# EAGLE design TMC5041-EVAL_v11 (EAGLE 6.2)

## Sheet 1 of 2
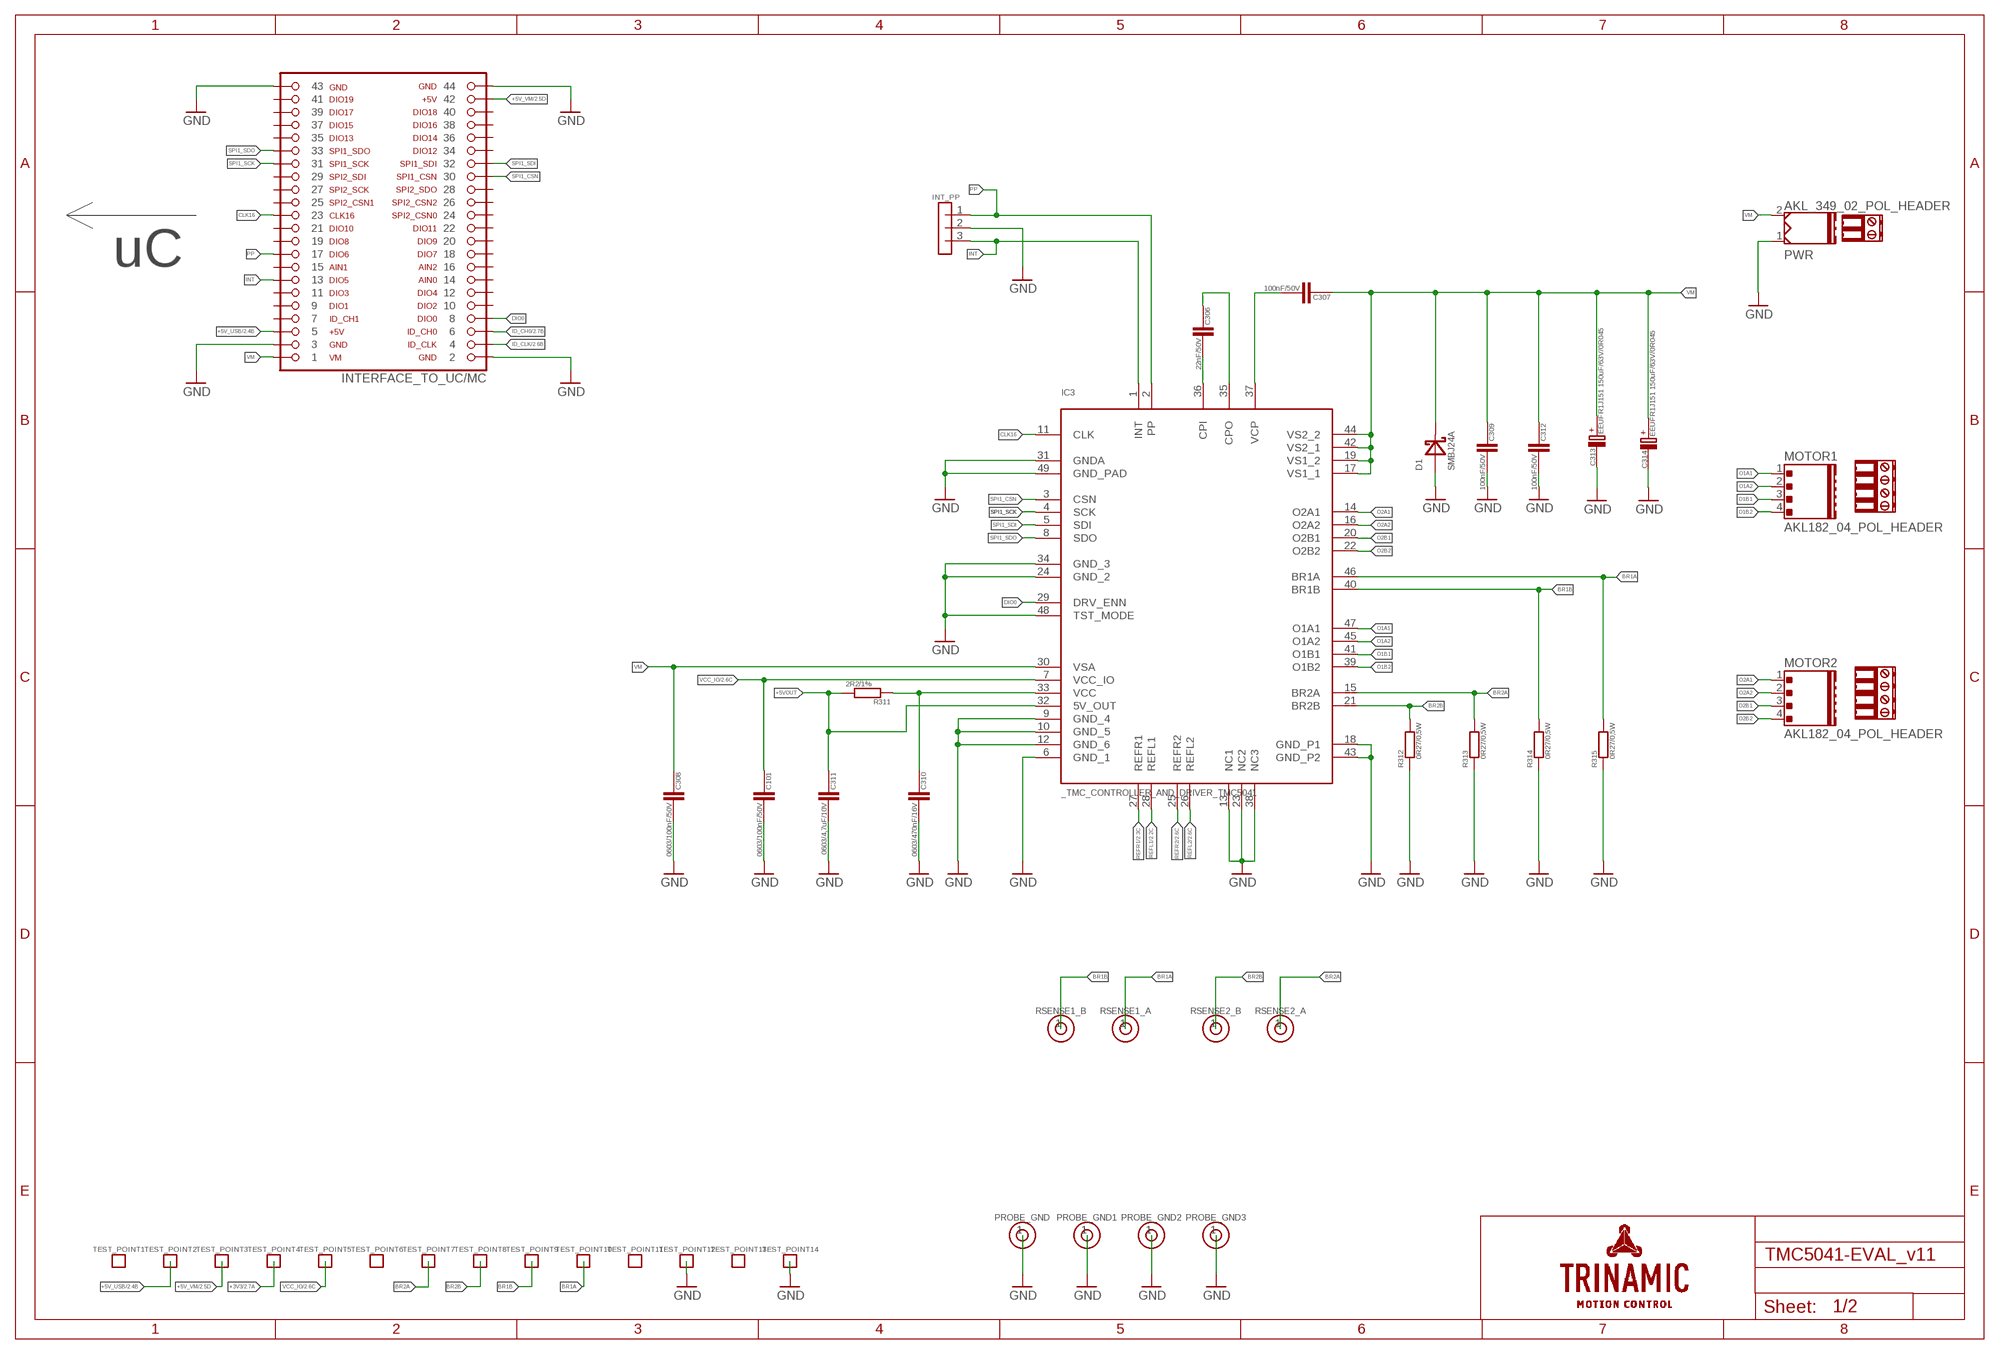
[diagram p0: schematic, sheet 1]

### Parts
C101  0603/100nF/50V  C/0603  [0603]
C306  22nF/50V  C/0603  [0603]
C307  100nF/50V  C/0603  [0603]
C308  0603/100nF/50V  C/0603  [0603]
C309  100nF/50V  C/0603  [0603]
C310  0603/470nF/16V  C/0603  [0603]
C311  0603/4,7uF/10V  C/0603  [0603]
C312  100nF/50V  C/0603  [0603]
C313  EEUFR1J151 150uF/63V/0R045  C_POL5X10X17.5  [C_POL_RAD_THT_5X10]
C314  EEUFR1J151 150uF/63V/0R045  C_POL5X10X17.5  [C_POL_RAD_THT_5X10]
D1  SMBJ24A  SMBJ  [SMB]
IC3  _TMC_CONTROLLER_AND_DRIVER_TMC5041  [_TMC_CONTROLLER_AND_DRIVER_QFN48]
INT_PP  MALE HEADER 2.54  3PIN_1ROWTHT  [3PIN_1ROW_2,54_THT]
INTERFACE_TO_UC/MC  FEMALE_HEADER_SMD_2.54_44_PINSHORTPADS_HOLES  [FEMALE_HEADER_SMD_254_44_PIN_SHORTPADS_HOLES]
MOTOR1  AKL182_04_POL_HEADER  [AKL169_04_POL]
MOTOR2  AKL182_04_POL_HEADER  [AKL169_04_POL]
PROBE_GND  NOT ASSEMBLED  1PIN_1ROW  [1PIN_1ROW_THT]
PROBE_GND1  NOT ASSEMBLED  1PIN_1ROW  [1PIN_1ROW_THT]
PROBE_GND2  NOT ASSEMBLED  1PIN_1ROW  [1PIN_1ROW_THT]
PROBE_GND3  NOT ASSEMBLED  1PIN_1ROW  [1PIN_1ROW_THT]
PWR  AKL_349_02_POL_HEADER  [AKL349_02_POL]
R311  2R2/1%  R/0603  [0603]
R312  0R27/0,5W  R  [1206]
R313  0R27/0,5W  R  [1206]
R314  0R27/0,5W  R  [1206]
R315  0R27/0,5W  R  [1206]
RSENSE1_A  NOT ASSEMBLED  1PIN_1ROW  [1PIN_1ROW_THT]
RSENSE1_B  NOT ASSEMBLED  1PIN_1ROW  [1PIN_1ROW_THT]
RSENSE2_A  NOT ASSEMBLED  1PIN_1ROW  [1PIN_1ROW_THT]
RSENSE2_B  NOT ASSEMBLED  1PIN_1ROW  [1PIN_1ROW_THT]
TERM1  AKL182_04_POL_TERMINAL  [EXTRA_TERMINAL]
TERM2  AKL182_04_POL_TERMINAL  [EXTRA_TERMINAL]
TERM3  AKL_330_2_POL_TERMINAL  [EXTRA_TERMINAL]
TEST_POINT1  NOT ASSEMBLED  PAD_ROUND  [PAD_R1.2]
TEST_POINT2  NOT ASSEMBLED  PAD_ROUND  [PAD_R1.2]
TEST_POINT3  NOT ASSEMBLED  PAD_ROUND  [PAD_R1.2]
TEST_POINT4  NOT ASSEMBLED  PAD_ROUND  [PAD_R1.2]
TEST_POINT5  NOT ASSEMBLED  PAD_ROUND  [PAD_R1.2]
TEST_POINT6  NOT ASSEMBLED  PAD_ROUND  [PAD_R1.2]
TEST_POINT7  NOT ASSEMBLED  PAD_ROUND  [PAD_R1.2]
TEST_POINT8  NOT ASSEMBLED  PAD_ROUND  [PAD_R1.2]
TEST_POINT9  NOT ASSEMBLED  PAD_ROUND  [PAD_R1.2]
TEST_POINT10  NOT ASSEMBLED  PAD_ROUND  [PAD_R1.2]
TEST_POINT11  NOT ASSEMBLED  PAD_ROUND  [PAD_R1.2]
TEST_POINT12  NOT ASSEMBLED  PAD_ROUND  [PAD_R1.2]
TEST_POINT13  NOT ASSEMBLED  PAD_ROUND  [PAD_R1.2]
TEST_POINT14  NOT ASSEMBLED  PAD_ROUND  [PAD_R1.2]

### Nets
+3V3: TEST_POINT4.P$1 ; also sheet 2
+5V_USB: INTERFACE_TO_UC/MC.5 TEST_POINT2.P$1 ; also sheet 2
+5V_VM: INTERFACE_TO_UC/MC.42 TEST_POINT3.P$1 ; also sheet 2
+5VOUT: C311.2 IC3.32(5V_OUT) R311.2
BR1A: IC3.46(BR1A) R315.2 RSENSE1_A.1 TEST_POINT10.P$1
BR1B: IC3.40(BR1B) R314.2 RSENSE1_B.1 TEST_POINT9.P$1
BR2A: IC3.15(BR2A) R313.2 RSENSE2_A.1 TEST_POINT7.P$1
BR2B: IC3.21(BR2B) R312.2 RSENSE2_B.1 TEST_POINT8.P$1
CLK16: IC3.11(CLK) INTERFACE_TO_UC/MC.23
CPI: C306.1 IC3.36(CPI)
CPO: C306.2 IC3.35(CPO)
DIO0: IC3.29(DRV_ENN) INTERFACE_TO_UC/MC.8
GND: C101.1 C308.1 C309.1 C310.1 C311.1 C312.1 C313.- C314.- D1.A IC3.6(GND_1) IC3.9(GND_4) IC3.10(GND_5) IC3.12(GND_6) IC3.13(NC1) IC3.18(GND_P1) IC3.23(NC2) IC3.24(GND_2) IC3.31(GNDA) IC3.34(GND_3) IC3.38(NC3) IC3.43(GND_P2) IC3.48(TST_MODE) IC3.49(GND_PAD) INT_PP.2 INTERFACE_TO_UC/MC.2 INTERFACE_TO_UC/MC.3 INTERFACE_TO_UC/MC.43 INTERFACE_TO_UC/MC.44 PROBE_GND1.1 PROBE_GND2.1 PROBE_GND3.1 PROBE_GND.1 PWR.1 R312.1 R313.1 R314.1 R315.1 TEST_POINT12.P$1 TEST_POINT14.P$1 ; also sheet 2
ID_CH0: INTERFACE_TO_UC/MC.6 ; also sheet 2
ID_CLK: INTERFACE_TO_UC/MC.4 ; also sheet 2
INT: IC3.1(INT) INT_PP.3 INTERFACE_TO_UC/MC.13
O1A1: IC3.47(O1A1) MOTOR1.1
O1A2: IC3.45(O1A2) MOTOR1.2
O1B1: IC3.41(O1B1) MOTOR1.3
O1B2: IC3.39(O1B2) MOTOR1.4
O2A1: IC3.14(O2A1) MOTOR2.1
O2A2: IC3.16(O2A2) MOTOR2.2
O2B1: IC3.20(O2B1) MOTOR2.3
O2B2: IC3.22(O2B2) MOTOR2.4
PP: IC3.2(PP) INT_PP.1 INTERFACE_TO_UC/MC.17
REFL1: IC3.28(REFL1) ; also sheet 2
REFL2: IC3.26(REFL2) ; also sheet 2
REFR1: IC3.27(REFR1) ; also sheet 2
REFR2: IC3.25(REFR2) ; also sheet 2
SPI1_CSN: IC3.3(CSN) INTERFACE_TO_UC/MC.30
SPI1_SCK: IC3.4(SCK) INTERFACE_TO_UC/MC.31
SPI1_SDI: IC3.5(SDI) INTERFACE_TO_UC/MC.32
SPI1_SDO: IC3.8(SDO) INTERFACE_TO_UC/MC.33
VCC: C310.2 IC3.33(VCC) R311.1
VCC_IO: C101.2 IC3.7(VCC_IO) TEST_POINT5.P$1 ; also sheet 2
VCP: C307.1 IC3.37(VCP)
VM: C307.2 C308.2 C309.2 C312.2 C313.+ C314.+ D1.C IC3.17(VS1_1) IC3.19(VS1_2) IC3.30(VSA) IC3.42(VS2_1) IC3.44(VS2_2) INTERFACE_TO_UC/MC.1 PWR.2
Unconnected: INTERFACE_TO_UC/MC.7 INTERFACE_TO_UC/MC.9 INTERFACE_TO_UC/MC.10 INTERFACE_TO_UC/MC.11 INTERFACE_TO_UC/MC.12 INTERFACE_TO_UC/MC.14 INTERFACE_TO_UC/MC.15 INTERFACE_TO_UC/MC.16 INTERFACE_TO_UC/MC.18 INTERFACE_TO_UC/MC.19 INTERFACE_TO_UC/MC.20 INTERFACE_TO_UC/MC.21 INTERFACE_TO_UC/MC.22 INTERFACE_TO_UC/MC.24 INTERFACE_TO_UC/MC.25 INTERFACE_TO_UC/MC.26 INTERFACE_TO_UC/MC.27 INTERFACE_TO_UC/MC.28 INTERFACE_TO_UC/MC.29 INTERFACE_TO_UC/MC.34 INTERFACE_TO_UC/MC.35 INTERFACE_TO_UC/MC.36 INTERFACE_TO_UC/MC.37 INTERFACE_TO_UC/MC.38 INTERFACE_TO_UC/MC.39 INTERFACE_TO_UC/MC.40 INTERFACE_TO_UC/MC.41 TEST_POINT1.P$1 TEST_POINT6.P$1 TEST_POINT11.P$1 TEST_POINT13.P$1

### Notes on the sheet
- uC

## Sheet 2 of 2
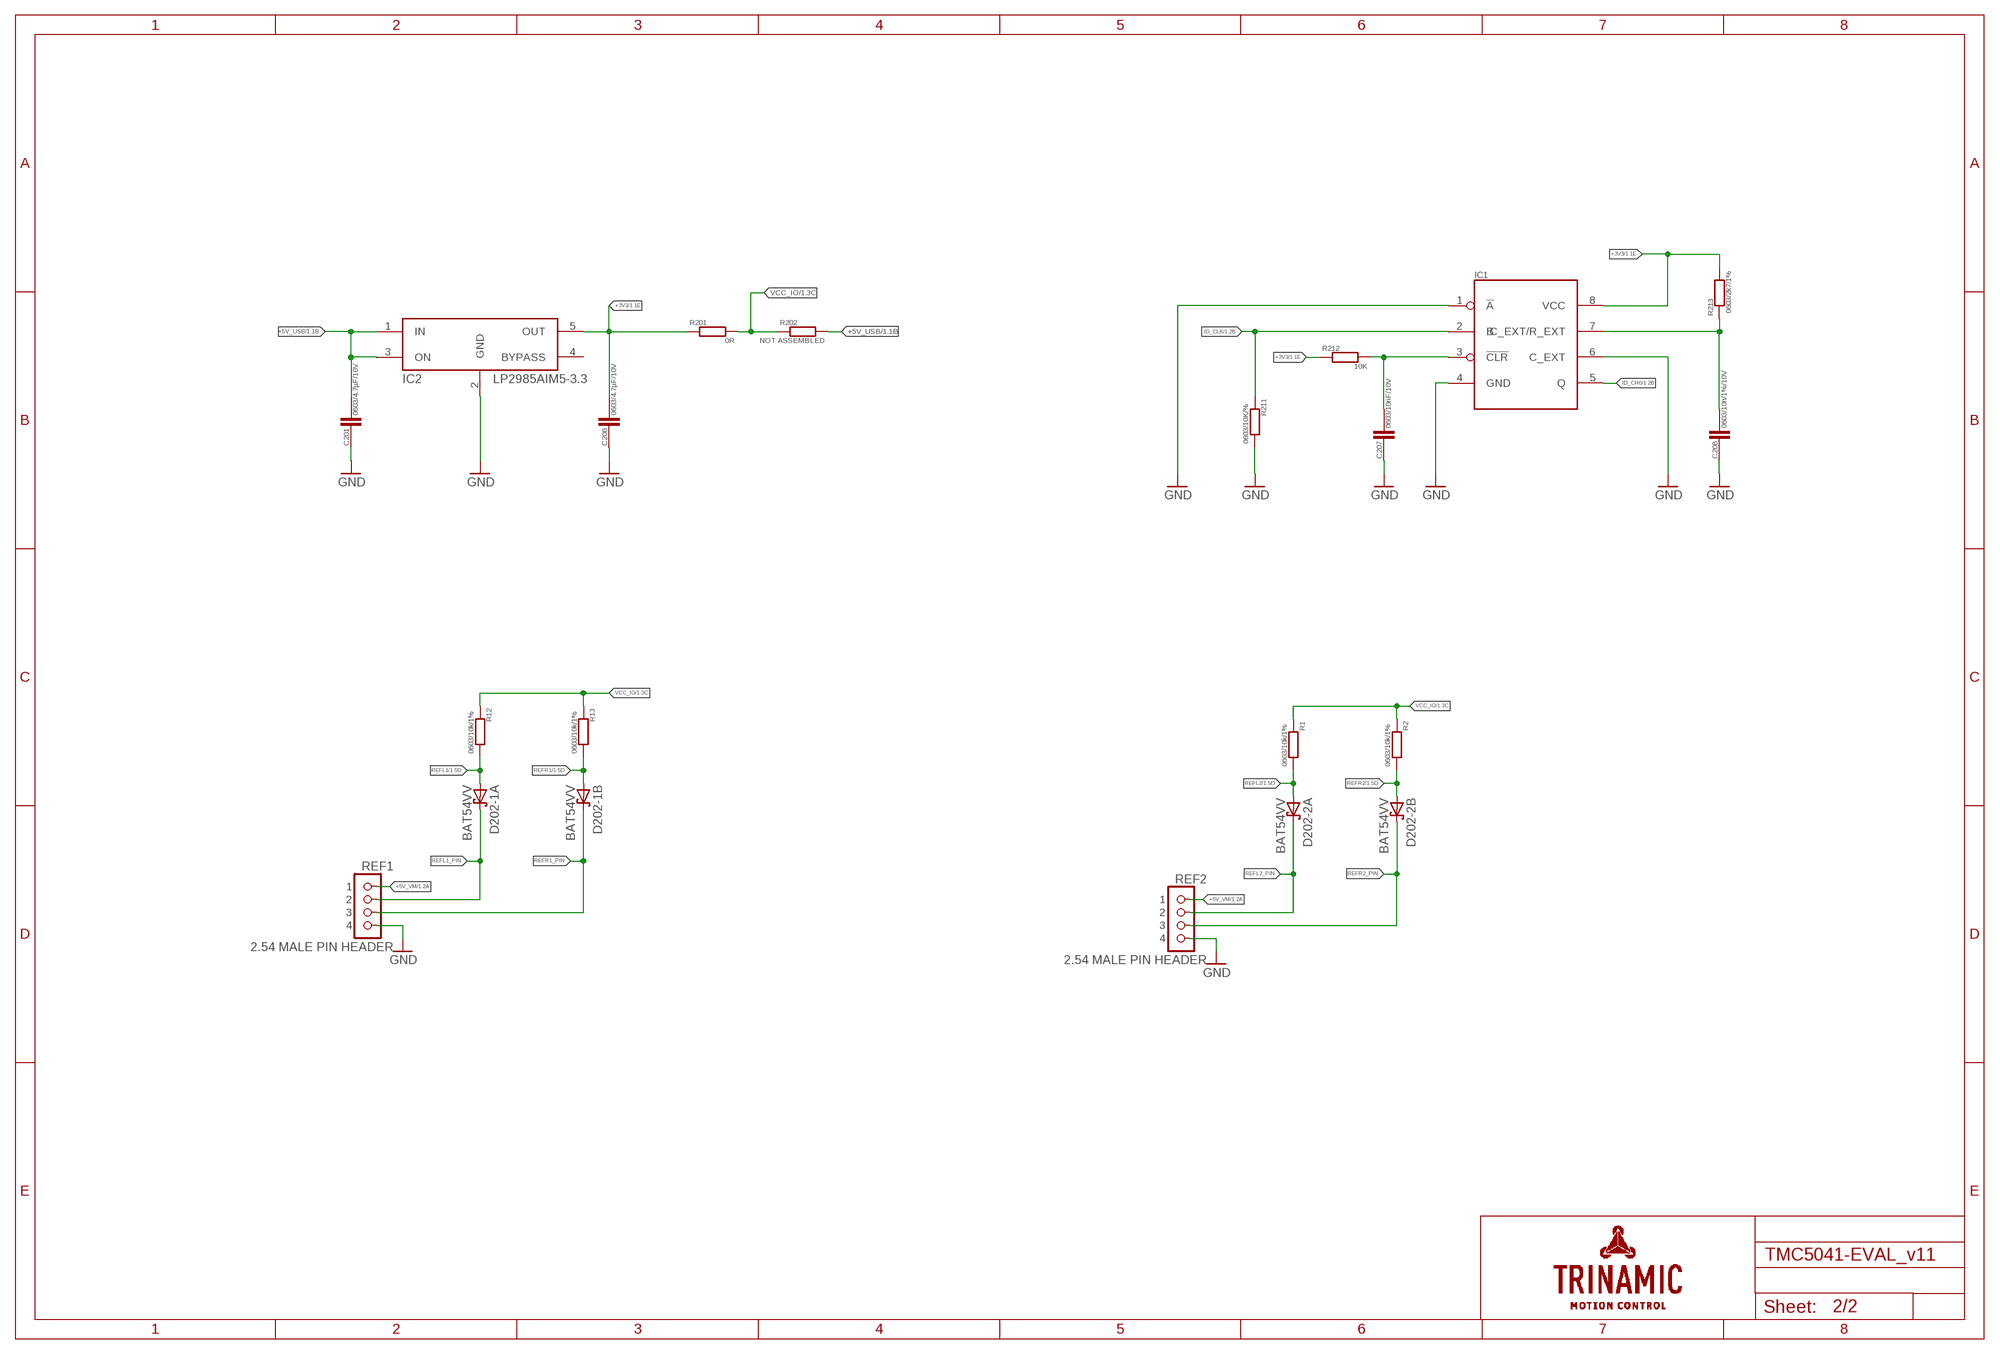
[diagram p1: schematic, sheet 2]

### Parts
C201  0603/4.7µF/10V  RCL_C/0603  [RCL_0603]
C206  0603/4.7µF/10V  RCL_C/0603  [RCL_0603]
C207  0603/10nF/10V  RCL_C/0603  [RCL_0603]
C208  0603/10n/1%/10V  RCL_C/0603  [RCL_0603]
D202-1  BAT54VV  BAS70VV  [SOT666]
D202-2  BAT54VV  BAS70VV  [SOT666]
IC1  SN74LVC1G123DCTR  [SN74LVC1G123DCTR]
IC2  LP2985AIM5-3.3  [SOT23-5]
R1  0603/10k/1%  R/0603  [0603]
R2  0603/10k/1%  R/0603  [0603]
R12  0603/10k/1%  R/0603  [0603]
R13  0603/10k/1%  R/0603  [0603]
R201  0R  R/0603  [0603]
R202  NOT ASSEMBLED  R/0603  [0603]
R211  0603/10K/%  RCL_R/0603  [RCL_0603]
R212  10K  RCL_R/0603  [RCL_0603]
R213  0603/2k7/1%  RCL_R/0603  [RCL_0603]
REF1  2.54 MALE PIN HEADER  4PIN_1ROWTHT  [4PIN_1ROW_2.54_THT]
REF2  2.54 MALE PIN HEADER  4PIN_1ROWTHT  [4PIN_1ROW_2.54_THT]

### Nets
+3V3: C206.1 IC1.8(VCC) IC2.5(OUT) R201.1 R212.1 R213.2 ; also sheet 1
+5V_USB: C201.1 IC2.1(IN) IC2.3(ON) R202.2 ; also sheet 1
+5V_VM: REF1.1 REF2.1 ; also sheet 1
GND: C201.2 C206.2 C207.2 C208.2 IC1.1(!A) IC1.4(GND) IC1.6(C_EXT) IC2.2(GND) R211.2 REF1.4 REF2.4 ; also sheet 1
ID_CH0: IC1.5(Q) ; also sheet 1
ID_CLK: IC1.2(B) R211.1 ; also sheet 1
N$1: C207.1 IC1.3(!CLR) R212.2
N$2: C208.1 IC1.7(C_EXT/R_EXT) R213.1
REFL1: D202-1.1(A:A) R12.2 ; also sheet 1
REFL1_PIN: D202-1.6(A:C) REF1.2
REFL2: D202-2.1(A:A) R1.2 ; also sheet 1
REFL2_PIN: D202-2.6(A:C) REF2.2
REFR1: D202-1.2(B:A) R13.2 ; also sheet 1
REFR1_PIN: D202-1.5(B:C) REF1.3
REFR2: D202-2.2(B:A) R2.2 ; also sheet 1
REFR2_PIN: D202-2.5(B:C) REF2.3
VCC_IO: R1.1 R2.1 R12.1 R13.1 R201.2 R202.1 ; also sheet 1
Unconnected: D202-1.3(C:A) D202-1.4(C:C) D202-2.3(C:A) D202-2.4(C:C) IC2.4(BYPASS)

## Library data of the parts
C101 C306-C312 = _TMC_TE_RCL:C
C201 C206-C208 = TMC_EVAL_driver_TE_v01:RCL_C
C313 C314 = _TMC_TE_RCL:C_POL
D1 = _TMC_TE_D:SMBJ
D202-1 D202-2 = diode:BAS70VV: Silicon Schottky Diodes General-purpose diode for high-speed switching Source: BAS70_1PS7XSB70_SER_8.pdf
IC1 = TMC_EVAL_driver_TE_v01:SN74LVC1G123DCTR
IC2 = TMC_EVAL_driver_TE_v01:LP2985AIM5-3.3
IC3 = TMC5041:_TMC_CONTROLLER_AND_DRIVER_TMC5041
INT_PP = _TMC_TE_con:3PIN_1ROW
INTERFACE_TO_UC/MC = _TMC_TE_con:FEMALE_HEADER_SMD_2.54_44_PIN; 1_PARTNUMBER: 098-3-044-1-NFX-YT0; 1_SUPPLIER: MPE Garry; 2_PARTNUMBER: HLE-122-02-F-DV; 2_SUPPLIER: Samtec
MOTOR1 MOTOR2 = _TMC_TE_con:AKL182_04_POL_HEADER: AKL header, shrouted, 4 pins; 1_PARTNUMBER: 31182104; 1_SUPPLIER: RIA CONNECT; 2_PARTNUMBER: AKL 182-04; 2_SUPPLIER: Reichelt
PROBE_GND PROBE_GND1-PROBE_GND3 RSENSE1_A RSENSE1_B RSENSE2_A RSENSE2_B = _TMC_TE_con:1PIN_1ROW
PWR = _TMC_TE_con:AKL_349_02_POL_HEADER: AKL header, shrouted, 2 pins; 1_PARTNUMBER: 31330102; 1_SUPPLIER: RIA CONNECT; 2_PARTNUMBER: AKL 330-02; 2_SUPPLIER: REICHELT
R1 R2 R12 R13 R201 R202 R311-R315 = _TMC_TE_RCL:R
R211-R213 = TMC_EVAL_driver_TE_v01:RCL_R
REF1 REF2 = _TMC_TE_con:4PIN_1ROW
TERM1 TERM2 = _TMC_TE_con:AKL182_04_POL_TERMINAL: AKL terminal, 4 pins; 1_PARTNUMBER: 31169104; 1_SUPPLIER: RIA CONNECT; 2_PARTNUMBER: AKL 169-04; 2_SUPPLIER: Reichelt
TERM3 = _TMC_TE_con:AKL_330_2_POL_TERMINAL: AKL terminal, 2 pins; 1_PARTNUMBER: 31349102; 1_SUPPLIER: RIA CONNECT; 2_PARTNUMBER: AKL 349-02; 2_SUPPLIER: Reichelt
TEST_POINT1-TEST_POINT14 = _TMC_TE_PADS:PAD_ROUND

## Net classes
0 default: width 0.254 mm, drill 0.15 mm

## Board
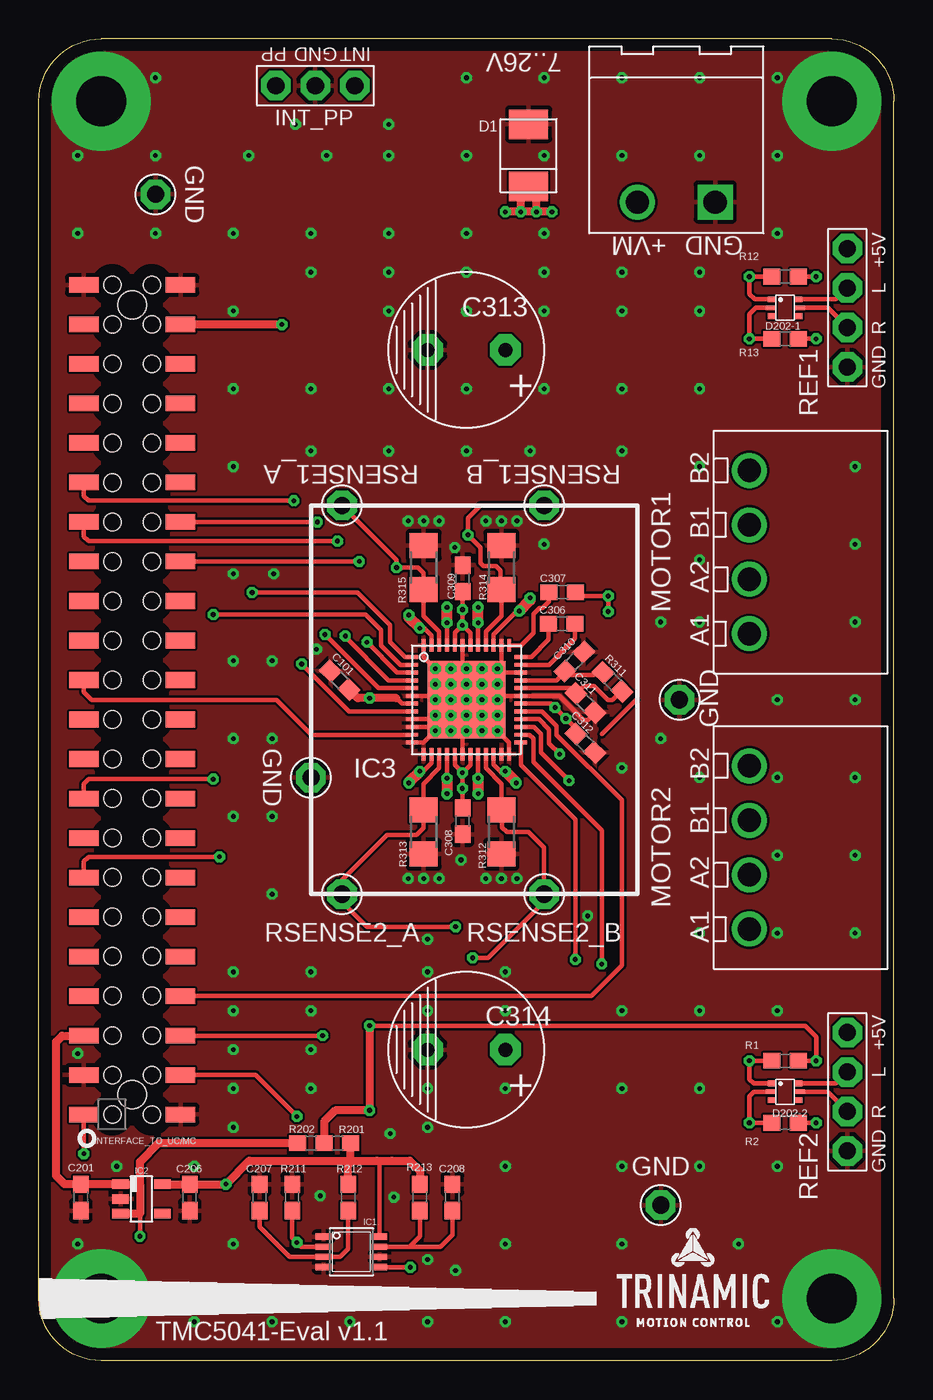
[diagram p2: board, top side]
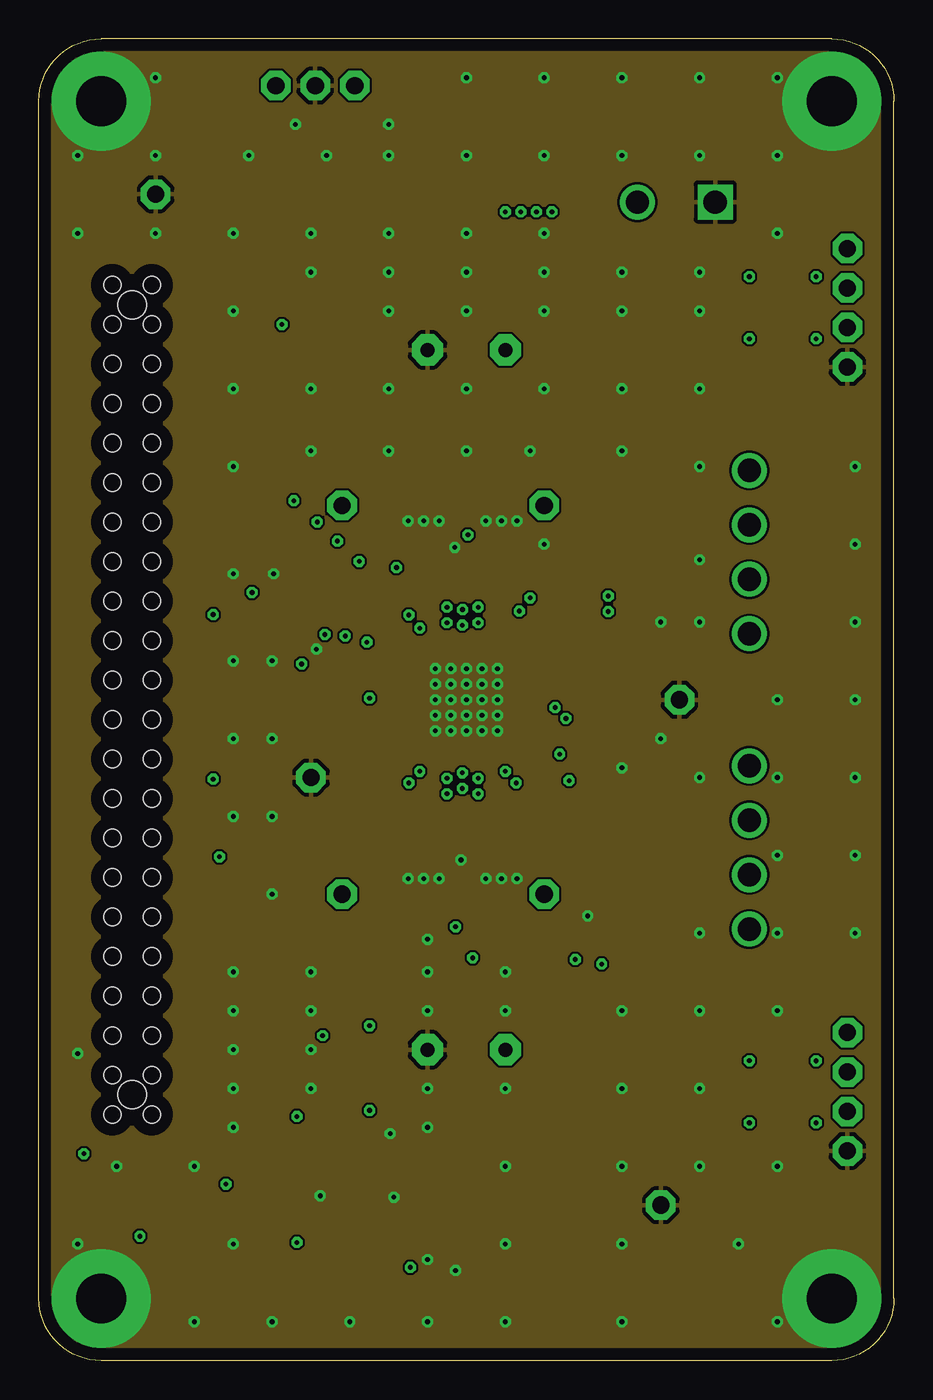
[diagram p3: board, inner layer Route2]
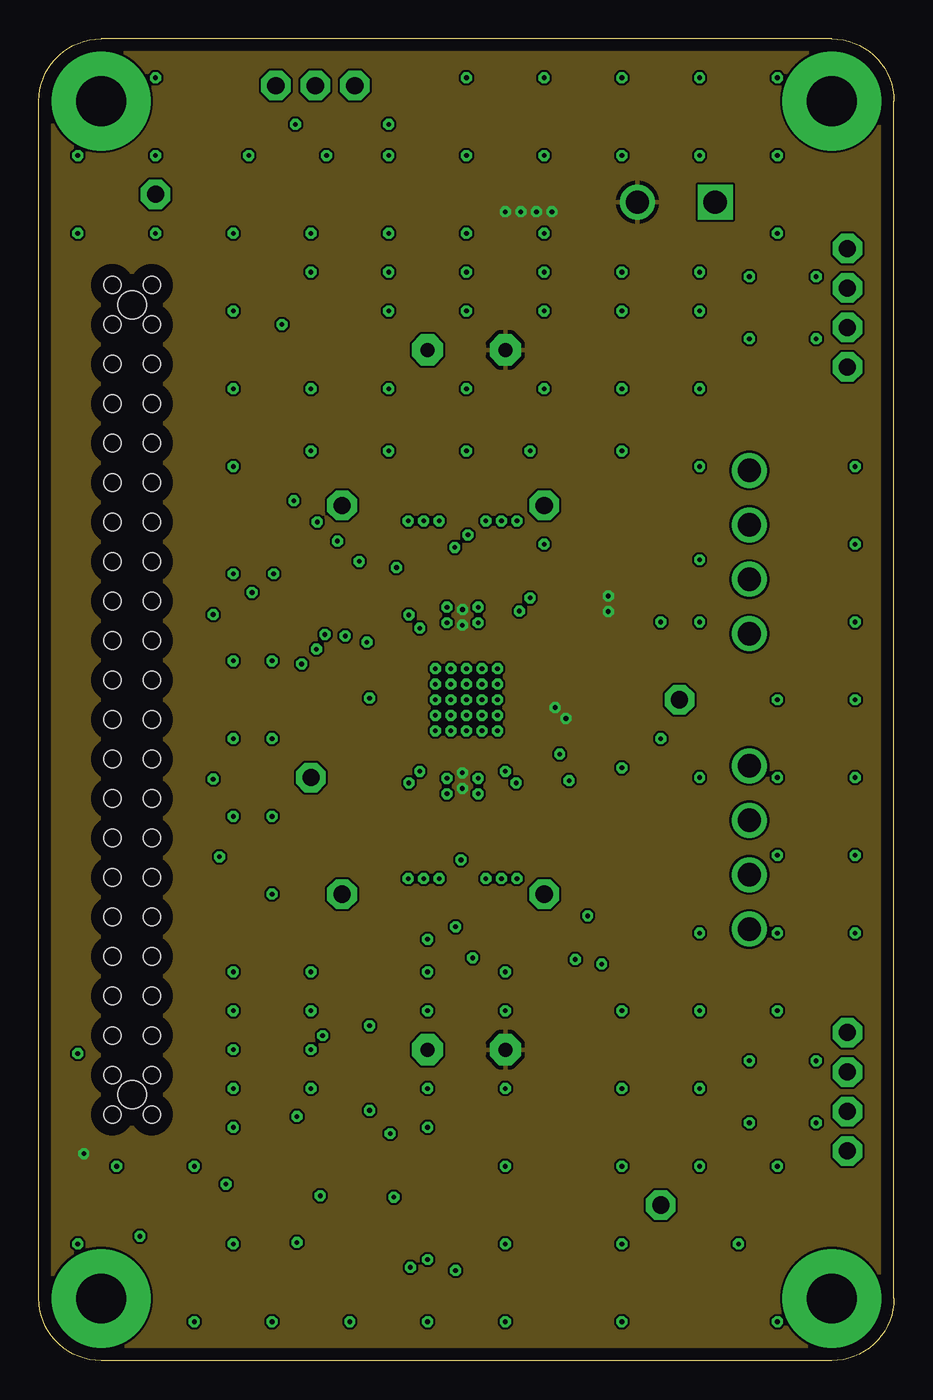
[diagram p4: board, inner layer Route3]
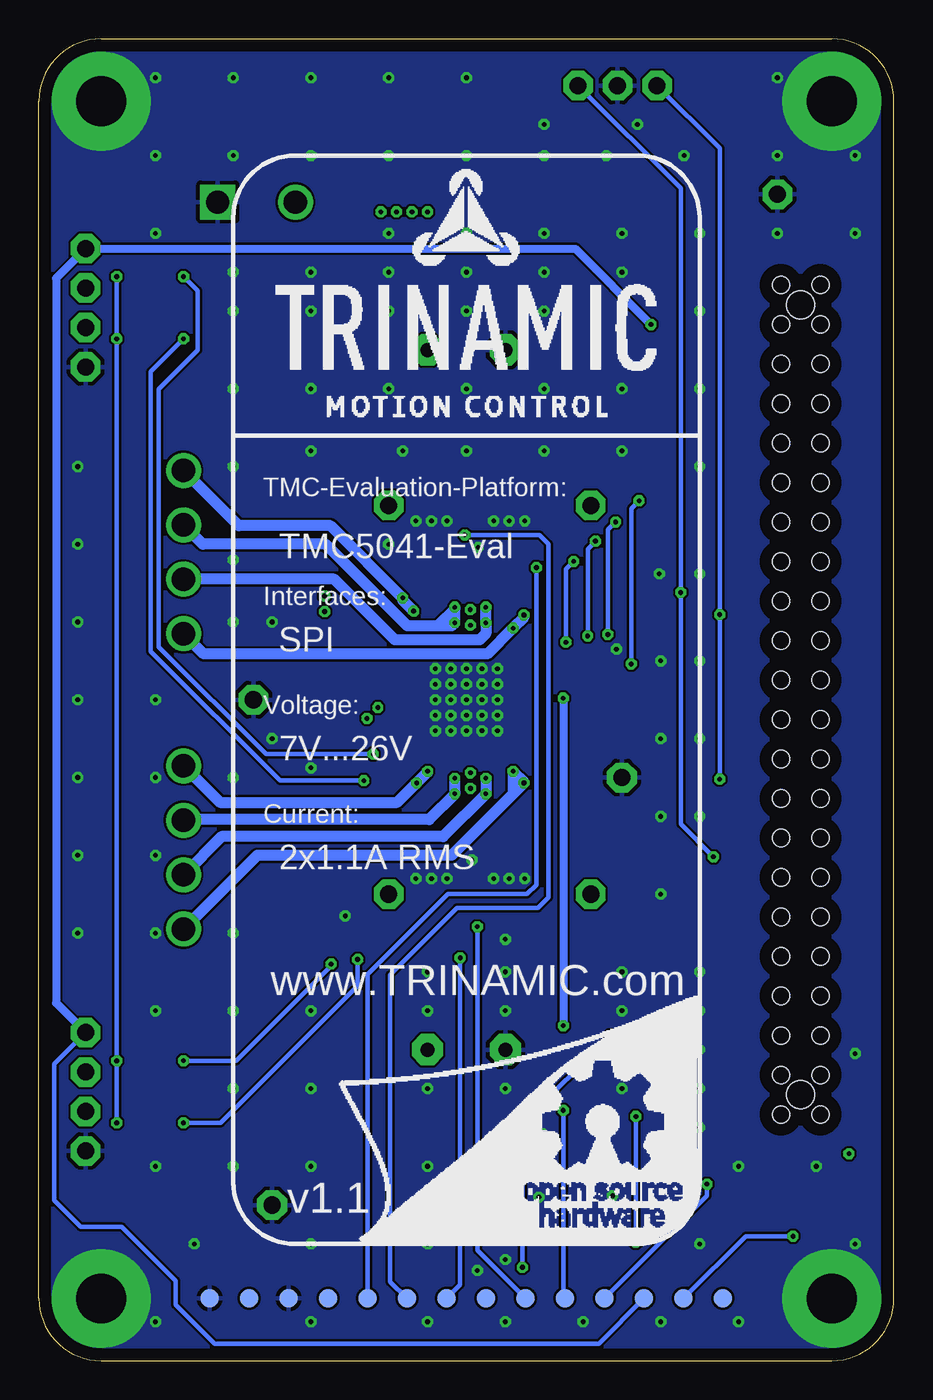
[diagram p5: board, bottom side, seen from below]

Size 55 x 85 mm. Coordinates in mm from the lower left corner, seen from the top.
Outline: 51,0 4,0 arc-90 0,4 0,81 arc-90 4,85 51,85 arc-90 55,81 55,4 arc-90 51,0
Copper layers (1*2*3*16): Top 0.018mm / dielectric 0.36mm / Route2 0.035mm / dielectric 0.71mm / Route3 0.035mm / dielectric 0.2mm / Bottom 0.018mm
Design rules: minimum track width 0.15mm, minimum drill 0.25mm, track to track 0.15mm, track to pad 0.15mm, pad to pad 0.1mm, via to via 0.15mm, smd to smd 0mil, copper to edge 0.8mm, drill to drill 8mil, minimum pad ring 10mil, minimum via ring 8mil, stop-mask expansion 4mil, vias tented up to drill 0.4mm, thermal gap 10mil

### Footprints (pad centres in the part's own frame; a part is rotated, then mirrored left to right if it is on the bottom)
0603 = smd 1.1 x 1: 1 -0.85,0; 2 0.85,0
RCL_0603 = smd 1.1 x 1: 1 -0.85,0; 2 0.85,0
C_POL_RAD_THT_5X10 = drill 0.9 pad 2 octagon: + 2.5,0; - -2.5,0
SMB = smd 1.9 x 2.5: A 2,0; C -2,0
SOT666 = smd 0.375 x 0.5: 1 -0.537,-0.85; 3 0.538,-0.85; 4 0.538,0.849; 6 -0.538,0.85 | smd 0.3 x 0.65: 2 0,-0.923; 5 0,0.925
SN74LVC1G123DCTR = smd 0.4 x 1: 1 -0.975,-1.8; 2 -0.325,-1.8; 3 0.325,-1.8; 4 0.975,-1.8; 5 0.975,1.8; 6 0.325,1.8; 7 -0.325,1.8; 8 -0.975,1.8
SOT23-5 = smd 0.6 x 1.05: 1 -0.95,-1.35; 2 0,-1.35; 3 0.95,-1.35; 4 0.95,1.35; 5 -0.95,1.35
_TMC_CONTROLLER_AND_DRIVER_QFN48 = smd 0.25 x 0.8: 1 -2.75,-3.5; 2 -2.25,-3.5; 3 -1.75,-3.5; 4 -1.25,-3.5; 5 -0.75,-3.5; 6 -0.25,-3.5; 7 0.25,-3.5; 8 0.75,-3.5; 9 1.25,-3.5; 10 1.75,-3.5; 11 2.25,-3.5; 12 2.75,-3.5; 25 2.75,3.5; 26 2.25,3.5; 27 1.75,3.5; 28 1.25,3.5; 29 0.75,3.5; 30 0.25,3.5; 31 -0.25,3.5; 32 -0.75,3.5; 33 -1.25,3.5; 34 -1.75,3.5; 35 -2.25,3.5; 36 -2.75,3.5 | smd 0.8 x 0.25: 13 3.5,-2.75; 14 3.5,-2.25; 15 3.5,-1.75; 16 3.5,-1.25; 17 3.5,-0.75; 18 3.5,-0.25; 19 3.5,0.25; 20 3.5,0.75; 21 3.5,1.25; 22 3.5,1.75; 23 3.5,2.25; 24 3.5,2.75; 37 -3.5,2.75; 38 -3.5,2.25; 39 -3.5,1.75; 40 -3.5,1.25; 41 -3.5,0.75; 42 -3.5,0.25; 43 -3.5,-0.25; 44 -3.5,-0.75; 45 -3.5,-1.25; 46 -3.5,-1.75; 47 -3.5,-2.25; 48 -3.5,-2.75 | smd 5 x 5: 49 0,0
3PIN_1ROW_2,54_THT = drill 1.1 pad 1.9 octagon: 1 -2.54,0; 2 0,0; 3 2.54,0
FEMALE_HEADER_SMD_254_44_PIN_SHORTPADS_HOLES = smd 1 x 1.9: 1 -26.67,3.11; 2 -26.67,-3.11; 3 -24.13,3.11; 4 -24.13,-3.11; 5 -21.59,3.11; 6 -21.59,-3.11; 7 -19.05,3.11; 8 -19.05,-3.11; 9 -16.51,3.11; 10 -16.51,-3.11; 11 -13.97,3.11; 12 -13.97,-3.11; 13 -11.43,3.11; 14 -11.43,-3.11; 15 -8.89,3.11; 16 -8.89,-3.11; 17 -6.35,3.11; 18 -6.35,-3.11; 19 -3.81,3.11; 20 -3.81,-3.11; 21 -1.27,3.11; 22 -1.27,-3.11; 23 1.27,3.11; 24 1.27,-3.11; 25 3.81,3.11; 26 3.81,-3.11; 27 6.35,3.11; 28 6.35,-3.11; 29 8.89,3.11; 30 8.89,-3.11; 31 11.43,3.11; 32 11.43,-3.11; 33 13.97,3.11; 34 13.97,-3.11; 35 16.51,3.11; 36 16.51,-3.11; 37 19.05,3.11; 38 19.05,-3.11; 39 21.59,3.11; 40 21.59,-3.11; 41 24.13,3.11; 42 24.13,-3.11; 43 26.67,3.11; 44 26.67,-3.11 | hole 1.8: -25.4,0; 25.4,0 | hole 1.1: -26.67,1.27; -24.13,1.27; -21.59,1.27; -19.05,1.27; -16.51,1.27; -13.97,1.27; -11.43,1.27; -8.89,1.27; -6.35,1.27; -3.81,1.27; -1.27,1.27; 1.27,1.27; 3.81,1.27; 6.35,1.27; 8.89,1.27; 11.43,1.27; 13.97,1.27; 16.51,1.27; 19.05,1.27; 21.59,1.27; 24.13,1.27; 26.67,1.27; -26.67,-1.27; -24.13,-1.27; -21.59,-1.27; -19.05,-1.27; -16.51,-1.27; -13.97,-1.27; -11.43,-1.27; -8.89,-1.27; -6.35,-1.27; -3.81,-1.27; -1.27,-1.27; 1.27,-1.27; 3.81,-1.27; 6.35,-1.27; 8.89,-1.27; 11.43,-1.27; 13.97,-1.27; 16.51,-1.27; 19.05,-1.27; 21.59,-1.27; 24.13,-1.27; 26.67,-1.27
AKL169_04_POL = drill 1.5: 1 -5.25,3.3; 2 -1.75,3.3; 3 1.75,3.3; 4 5.25,3.3
1PIN_1ROW_THT = drill 1.1 pad 1.9 octagon: 1 0,0
AKL349_02_POL = drill 1.5 square: 1 -2.5,4 | drill 1.5: 2 2.5,4
1206 = smd 1.6 x 1.803: 1 -1.422,0; 2 1.422,0
4PIN_1ROW_2.54_THT = drill 1.1 pad 1.9 octagon: 1 -3.81,0; 2 -1.27,0; 3 1.27,0; 4 3.81,0
PAD_R1.2 = smd 1.2 x 1.2: P$1 0,0

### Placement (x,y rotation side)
C101  19.35,43.76 315 top
C201  2.7,10.5 270 top
C206  9.7,10.5 270 top
C207  14.2,10.5 90 top
C208  26.6,10.5 90 top
C306  33.63,47.38 0 top
C307  33.66,49.42 0 top
C308  27.25,34.7 90 top
C309  27.25,50.3 270 top
C310  34.44,44.96 225 top
C311  35.15,42.3 135 top
C312  35.15,39.7 135 top
C313  27.5,65 0 top
C314  27.5,20 0 top
D1  31.5,77.5 90 top
D202-1  48,67.71 270 top
D202-2  48,17.29 270 top
IC1  20.1,7 270 top
IC2  6.6,10.4 270 top
IC3  27.5,42.5 270 top
INT_PP  17.78,82 0 top
INTERFACE_TO_UC/MC  6,42.5 90 top
MOTOR1  49,52 90 top
MOTOR2  49,33 90 top
PROBE_GND  41.2,42.5 0 top
PROBE_GND1  17.5,37.5 180 top
PROBE_GND2  7.5,75 270 top
PROBE_GND3  40,10 0 top
PWR  41,78.5 180 top
R1  48,19.29 180 top
R2  48,15.29 180 top
R12  48,69.71 180 top
R13  48,65.71 180 top
R201  19.2,14 180 top
R202  17.5,14 180 top
R211  16.3,10.5 90 top
R212  19.9,10.5 270 top
R213  24.5,10.5 90 top
R311  36.9,43.65 315 top
R312  29.75,34 90 top
R313  24.75,34 90 top
R314  29.75,51 270 top
R315  24.75,51 270 top
REF1  52,67.71 270 top
REF2  52,17.29 270 top
RSENSE1_A  19.5,55 0 top
RSENSE1_B  32.5,55 0 top
RSENSE2_A  19.5,30 0 top
RSENSE2_B  32.5,30 0 top
TERM1  -1,-1.1 0 top
TERM2  -2,-2.2 0 top
TERM3  not placed on the board
TEST_POINT1  11,4 0 bottom
TEST_POINT2  13.54,4 0 bottom
TEST_POINT3  16.08,4 0 bottom
TEST_POINT4  18.62,4 0 bottom
TEST_POINT5  21.16,4 0 bottom
TEST_POINT6  26.24,4 0 bottom
TEST_POINT7  23.7,4 0 bottom
TEST_POINT8  28.78,4 0 bottom
TEST_POINT9  31.32,4 0 bottom
TEST_POINT10  33.86,4 0 bottom
TEST_POINT11  36.4,4 0 bottom
TEST_POINT12  38.94,4 0 bottom
TEST_POINT13  41.48,4 0 bottom
TEST_POINT14  44.02,4 0 bottom
U$1  [TMC_EVAL_RIGHT_BAR]  0,0 0 top
U$3  [TMC_EVAL_BACK_NO_DOCU]  55,0 0 bottom

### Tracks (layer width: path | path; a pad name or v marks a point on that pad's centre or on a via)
+3V3  (via drill 0.3 pad 0.3)
  Top 0.3: 23,12.85 22.7,12.85 | IC1.8 21.9,12.7 21.75,12.85
  Top 0.5: IC2.5 C206.1 v12.03,11.35 13.53,12.85 19.9,12.85 | 19.9,12.85 21.75,12.85 22.7,12.85 23.85,12.85 24.5,12.2 R213.2 | R212.1 19.9,12.85 | 19.9,12.85 20.05,13 R201.1
  Bottom 0.3: v12.03,11.35 12.03,10.59 TEST_POINT4.P$1
+5V_USB  (via drill 0.3 pad 0.3)
  Top 0.3: 6.5,9.45 v6.5,8
  Top 0.5: 2.51,20.91 INTERFACE_TO_UC/MC.5 1.5,20.9 1.1,20.5 1.1,11.9 1.65,11.35 C201.1 IC2.1 6.5,11.35 | 6.5,11.35 6.5,9.45 IC2.3 | 6.5,11.35 6.5,12.8 7.7,14 R202.2
  Bottom 0.3: v6.5,8 9.54,8 TEST_POINT2.P$1
+5V_VM  (via drill 0.3 pad 0.3)
  Top 0.5: v15.63,66.63 INTERFACE_TO_UC/MC.42
  Bottom 0.3: TEST_POINT3.P$1 18.98,1.1 43.7,1.1 46.2,3.6 46.2,5.12 49.68,8.6 52.3,8.6 54,10.3 54,19.1 REF2.1
  Bottom 0.5: REF2.1 53.9,23 53.9,69.6 52,71.5 REF1.1 51.98,71.5 20.5,71.5 v15.63,66.63
+5VOUT
  Top 0.3: IC3.32 34.2,43.25 C311.2 35.05,43.4 35.7,43.4 36.6,42.5 36.9,42.5 37.45,43.05 R311.2
BR1A  (via drill 0.3 pad 0.3)
  Top 0.3: IC3.46 25.75,46.9 24.75,47.9 R315.2 24.75,50.65 24.4,51 v23,51 23,51.5 RSENSE1_A.1
  Bottom 0.3: v23,51 23,30.6 23.6,30 28.7,30 33.86,24.84 TEST_POINT10.P$1 33.8,4.06
BR1B  (via drill 0.3 pad 0.3)
  Top 0.3: IC3.40 28.75,46.9 29.75,47.9 R314.2 29.32,49.58 29.32,49.78 29.58,49.78 29.7,49.9 29.7,50.8 29.4,51.1 28.6,51.1 28.4,51.3 28.4,52.3 v27.6,53.1 27.6,54.2 28.4,55 RSENSE1_B.1
  Bottom 0.3: v27.6,53.1 22.8,53.1 22.22,52.52 22.22,29.78 22.9,29.1 28.1,29.1 32.4,24.8 32.4,5.08 TEST_POINT9.P$1
BR2A  (via drill 0.3 pad 0.3)
  Top 0.3: IC3.15 25.75,38.1 24.75,37.1 R313.2 24.75,34.25 24.3,33.8 22.4,33.8 19.5,30.9 RSENSE2_A.1 19.5,29.5 21.1,27.9 v26.8,27.9
  Bottom 0.3: TEST_POINT7.P$1 26.8,7.1 v26.8,27.9
BR2B  (via drill 0.3 pad 0.25)
  Top 0.3: IC3.21 28.75,38.1 29.75,37.1 R312.2 29.75,35.25 29.8,35.2 29.8,34.3 30.1,34 31.5,34 32.5,33 RSENSE2_B.1 32.5,29.5 28.9,25.9 v27.9,25.9
  Bottom 0.3: 28.8,4.02 TEST_POINT8.P$1 27.9,4.88 v27.9,25.9
CLK16
  Top 0.3: IC3.11 17.55,40.25 15.3,42.5 3.4,42.5 2.89,43.01 INTERFACE_TO_UC/MC.23
CPI
  Top 0.3: IC3.36 31.67,45.25 32.78,46.37 C306.1
CPO
  Top 0.3: IC3.35 32.81,44.75 34.48,46.42 C306.2
DIO0
  Top 0.3: IC3.29 32.35,41.75 33.3,40.8 33.3,40.25 37.5,36.05 37.5,34.07 37.51,34.06 37.51,25.41 35.55,23.45 INTERFACE_TO_UC/MC.8
GND  (via drill 0.3 pad 0.3, 3.2 pad 6.35)
  Top 0.3: IC3.6 25.15,42.75 25.2,42.7 27.3,42.7 IC3.49 | IC3.18 27.25,42.25 IC3.49 | IC3.43 27.25,42.75 IC3.49 | IC3.34 29.25,44.25 IC3.49 | IC3.24 30.25,39.75 IC3.49 | v26.5,43.5 26.5,42.75 IC3.31 33.47,42.75 35.02,41.2 35.3,41.2 35.75,41.65 C311.1 | IC3.48 24.75,45.25 v25.5,44.5 | IC3.10 25.25,40.75 v25.5,40.5 24.75,39.75 IC3.12 | IC3.9 26.25,41.25 IC3.49 | IC3.38 29.75,44.75 v29.5,44.5
  other vias: 26.5,44.5 25.5,42.5 25.5,43.5 26.5,40.5 27.5,40.5 29.5,40.5 25.5,41.5 28.5,40.5 29.5,43.5 28.5,44.5 27.5,44.5 29.5,42.5 29.5,41.5 27.5,41.5 26.5,42.5 27.5,42.5 28.5,42.5 27.5,43.5 23.75,54 24.75,54 25.75,54 28.75,54 29.75,54 30.75,54 23.75,31 24.75,31 25.75,31 29.75,31 30.75,31 28.75,31 37.5,58.5 26.5,41.5 28.5,41.5 28.5,43.5 27.15,32.2 26.75,52.3 4,4 51,4 51,81 4,81 32.5,82.5 37.5,82.5 42.5,82.5 47.5,82.5 47.5,77.5 42.5,77.5 37.5,77.5 32.5,77.5 27.5,77.5 27.5,82.5 18.5,77.5 7.5,77.5 2.5,77.5 2.5,72.5 7.5,72.5 12.5,72.5 37.5,62.5 42.5,67.5 42.5,57.5 52.5,57.5 31.6,58.5 27.5,58.5 17.5,58.5 32.5,52.5 52.5,52.5 52.5,47.5 52.5,42.5 40,47.5 42.5,47.5 52.5,37.5 42.5,37.5 40,40 52.5,32.5 52.5,27.5 37.5,17.5 15,35 30,12.5 17.5,20 12.5,20 37.5,12.5 47.5,12.5 37.5,7.5 30,7.5 12.5,7.5 2.5,7.5 30,2.5 37.5,2.5 47.5,2.5 25,2.5 20,2.5 12.5,22.5 25,15 17.5,62.5 17.5,72.5 22.5,70 32.5,67.5 32.5,62.5 47.5,42.5 17.85,45.75 42.5,62.5 27.5,72.5 27.5,67.5 27.5,62.5 22.5,67.5 22.5,58.5 22.5,62.5 17.5,17.5 12.5,17.5 25,17.5 30,17.5 26.8,5.8 25,6.5 18.1,10.6 22.6,14.6 37.5,22.5 42.5,27.5 5,12.5 10,12.5 42.5,51.5 22.5,79.5 16.5,79.5 7.5,82.5 32.5,72.5 37.5,67.5 42.5,70 25,27.1 17.5,25 12.5,50.6 15,45 12.5,57.5 42.5,12.5 27.5,70 32.5,70 37.5,70 17.5,22.5 12.5,62.5 22.84,10.51 35.3,28.6 12.5,15 15,40 13.5,77.5 22.5,77.5 22.5,72.5 17.5,70 47.5,72.5 42.5,22.5 47.5,22.5 42.5,17.5 15,2.5 10,2.5 2.5,19.75 37.5,38.12 25,25 30,25 12.5,35 15,30 45,7.5 25,22.5 30,22.5 12.5,25 47.5,37.5 47.5,32.5 47.5,27.5 12.5,67.5 15.1,50.6 12.5,45 12.5,40
  pour Top: 0,85 55,85 55,0 0,0
  pour Bottom: 0.2,85 55,85 55,0 0,0
  pour Route2: 0,85 55,85 55,0 0,0
ID_CH0  (via drill 0.3 pad 0.3)
  Top 0.3: 8.61,20.9 8.9,20.9 v18.25,20.9 | IC1.5 21.93,6 v23.9,6
  Top 0.5: INTERFACE_TO_UC/MC.6 8.9,20.9
  Bottom 0.3: v23.9,6 23.9,15.25 v18.25,20.9
ID_CLK  (via drill 0.3)
  Top 0.3: R211.1 16.3,7.9 v16.6,7.6 16.88,7.33 IC1.2 | INTERFACE_TO_UC/MC.4 13.93,18.37 v16.6,15.7
  Bottom 0.3: v16.6,7.6 v16.6,15.7
INT  (via drill 0.3 pad 0.3)
  Top 0.3: INTERFACE_TO_UC/MC.13 2.89,32.09 3.2,32.4 v11.61,32.4 | IC3.1 23.55,45.25 22.6,46.2 22.6,47.3 20.5,49.4 v13.71,49.4
  Bottom 0.3: v11.61,32.4 13.71,34.5 v13.71,49.4 13.71,75.39 INT_PP.3
N$1
  Top 0.3: C207.1 14.2,8.6 16.12,6.67 IC1.3 19.38,6.67 19.9,7.2 R212.2
N$2
  Top 0.3: R213.1 24.5,8 23.82,7.33 | IC1.7 23.82,7.33 | C208.1 26.6,8.1 25.82,7.33 23.82,7.33
N$9
  Top 0.3: 38.4,42.5 36.2,40.3
O1A1  (via drill 0.3 pad 0.3)
  Top 0.3: IC3.47 25.25,46.62 23.92,47.95 v23.8,47.95
  Top 0.7: v24.5,47.1 23.8,47.8 v23.8,47.95
  Bottom 0.7: v23.8,47.95 23.8,47.8 v24.5,47.1 26.15,45.45 44.4,45.45 MOTOR1.1
O1A2  (via drill 0.3 pad 0.3)
  Top 0.3: IC3.45 v26.25,47.45
  Top 0.7: v26.25,47.45 v26.25,48.45
  Bottom 0.7: MOTOR1.2 36,50.25 32.1,46.35 26.65,46.35 26.25,46.75 v26.25,47.45 v26.25,48.45
O1B1  (via drill 0.3 pad 0.3)
  Top 0.3: IC3.41 v28.25,47.45
  Top 0.7: v28.25,47.45 v28.25,48.45
  Bottom 0.7: MOTOR1.3 44.45,52.5 36.55,52.5 31.3,47.25 28.45,47.25 v28.25,47.45 v28.25,48.45 28.25,48.35 29.3,47.3
O1B2  (via drill 0.3 pad 0.3)
  Top 0.3: IC3.39 29.25,46.7 v31.6,49.05
  Top 0.7: v30.9,48.2 31.6,48.9 31.6,49
  Bottom 0.7: MOTOR1.4 42.15,53.7 36.25,53.7 v31.6,49.05 31.6,48.9 v30.9,48.2
O2A1  (via drill 0.3 pad 0.3)
  Top 0.3: IC3.14 25.25,38.45 23.95,37.15 v23.8,37.15
  Top 0.7: v24.5,37.9 23.8,37.2 v23.8,37.15
  Bottom 0.7: MOTOR2.1 40.95,32.5 28.45,32.5 24.57,36.38 24.5,36.45 | 24.5,36.45 v23.8,37.15 | 23.8,37.2 v24.5,37.9 24.5,36.45
O2A2  (via drill 0.3 pad 0.3)
  Top 0.3: IC3.16 v26.25,37.45
  Top 0.7: v26.25,37.45 v26.25,36.45
  Bottom 0.7: v26.25,37.45 v26.25,36.45 29,33.7 43.25,33.7 MOTOR2.2
O2B1  (via drill 0.3 pad 0.3)
  Top 0.3: IC3.20 v28.25,37.45
  Top 0.7: v28.25,37.45 v28.25,36.45
  Bottom 0.7: 28.25,36.6 v28.25,36.45 | v28.25,36.45 v28.25,37.45 | v28.25,36.45 29.9,34.8 45.65,34.8 MOTOR2.3
O2B2  (via drill 0.3 pad 0.3)
  Top 0.3: IC3.22 29.25,38.35 30.45,37.15 v30.7,37.15
  Top 0.7: v30,37.9 30.7,37.2 v30.7,37.15
  Bottom 0.7: MOTOR2.4 43.35,35.9 31.95,35.9 v30.7,37.15 | v30,37.9 30,37.84 v30.7,37.14
PP  (via drill 0.3 pad 0.3)
  Top 0.3: INTERFACE_TO_UC/MC.17 2.89,37.09 3.2,37.4 v11.21,37.4 | IC3.2 23.25,44.75 22,46 22,47 21.02,47.98 v11.21,47.98
  Bottom 0.3: v11.21,37.4 v11.21,47.98 11.21,77.97 INT_PP.1
REFL1  (via drill 0.3 pad 0.3)
  Top 0.3: IC3.28 32.15,41.25 32.8,40.6 32.8,39.7 v33.5,39 | R12.2 v45.7,69.71 45.7,68.6 46.05,68.25 D202-1.1
  Bottom 0.3: v33.5,39 40.4,39 47.3,45.9 47.3,62.49 44.8,64.99 44.8,68.81 v45.7,69.71
REFL1_PIN
  Top 0.3: D202-1.6 51.27,68.25 REF1.2
REFL2  (via drill 0.3 pad 0.3)
  Top 0.3: IC3.26 31.55,40.25 31.8,40 31.8,38.5 36.2,34.1 v36.2,25.5 | D202-2.1 45.97,17.83 45.7,18.1 v45.7,19.29 R1.2
  Bottom 0.3: v36.2,25.5 36.2,25.39 42.3,19.29 v45.7,19.29
REFL2_PIN
  Top 0.3: D202-2.6 51.27,17.83 REF2.2
REFR1  (via drill 0.3 pad 0.3)
  Top 0.3: IC3.27 31.85,40.75 32.3,40.3 32.3,39.1 v34.1,37.3 | R13.2 v45.7,65.71 45.7,67.3 46.11,67.71 D202-1.2
  Bottom 0.3: v34.1,37.3 39.5,37.3 47.8,45.6 47.8,63.61 v45.7,65.71
REFR1_PIN
  Top 0.3: D202-1.5 50.73,67.71 REF1.3
REFR2  (via drill 0.3 pad 0.3)
  Top 0.3: IC3.25 31,38.3 34.5,34.8 v34.5,25.8 | R2.2 v45.7,15.29 45.7,17 45.99,17.29 D202-2.2
  Bottom 0.3: v34.5,25.8 34.5,24.1 43.31,15.29 v45.7,15.29
REFR2_PIN
  Top 0.3: D202-2.5 50.73,17.29 REF2.3
SPI1_CSN  (via drill 0.3 pad 0.3)
  Top 0.3: v20.6,51.4 INTERFACE_TO_UC/MC.30 | IC3.3 23.05,44.25 v21.1,46.2
  Bottom 0.3: v21.1,46.2 21.1,50.9 v20.6,51.4
SPI1_SCK  (via drill 0.3 pad 0.3)
  Top 0.3: INTERFACE_TO_UC/MC.31 2.89,53.01 3.2,52.7 v19.2,52.7 | IC3.4 22.5,43.75 19.65,46.6 v19.7,46.6
  Bottom 0.3: v19.7,46.6 19.7,52.2 v19.2,52.7
SPI1_SDI  (via drill 0.3 pad 0.25)
  Top 0.3: INTERFACE_TO_UC/MC.32 v17.9,53.93 | IC3.5 21.85,43.25 v18.4,46.7
  Bottom 0.3: v18.4,46.7 18.4,53.43 v17.9,53.93
SPI1_SDO  (via drill 0.3 pad 0.3)
  Top 0.3: INTERFACE_TO_UC/MC.33 2.89,55.61 3.2,55.3 v16.4,55.3 | IC3.8 19.95,41.75 v16.9,44.8
  Bottom 0.3: v16.9,44.8 16.9,54.8 v16.4,55.3
VCC
  Top 0.3: IC3.33 33.28,43.75 33.84,44.31 C310.2 arc90 34.1,44.1 35.7,44.1 arc-90 35.85,44.25 R311.1
VCC_IO  (via drill 0.3 pad 0.3)
  Top 0.3: IC3.7 23.35,42.25 23,42.6 | R12.1 v49.99,69.71 | v49.99,65.71 R13.1 | v49.99,15.29 R2.1 | R1.1 v49.99,19.28 49.99,20.84 49.29,21.54 v21.27,21.54
  Top 0.5: 23,42.6 v21.27,42.6 20.5,42.6 C101.2 | v21.27,21.54 v21.27,16.09 19.06,16.09 18.35,15.38 R202.1
  Bottom 0.3: v21.27,16.09 21.27,4.11 TEST_POINT5.P$1 | v49.99,69.71 v49.99,65.71 v49.99,19.28 v49.99,15.29
  Bottom 0.5: v21.27,42.6 v21.27,21.54
VCP
  Top 0.3: IC3.37 31,46 31.8,46.8 31.8,48 32.2,48.4 32.4,48.4 32.81,48.81 C307.1
VM  (via drill 0.3 pad 0.3)
  Top 0.3: C308.2 v27.25,37.79 v27.24,37.8 | IC3.17 26.75,38.29 v27.24,37.8 | IC3.19 27.75,38.31 v27.24,37.8 | INTERFACE_TO_UC/MC.1 v2.89,13.31 | IC3.30 32.95,42.25 v33.2,42 v33.9,41.3 34.9,40.3 C312.2 | v36.62,48.17 v36.62,49.17 34.67,49.17 34.52,49.32 C307.2 | IC3.44 26.75,46.81 v27.24,47.3 | IC3.42 27.75,46.79 v27.24,47.3 | v27.24,47.3 v27.24,48.29 v27.25,48.3 C309.2
  Top 0.5: v33,73.88 v32,73.88 | v32,73.88 v31,73.88 | v31,73.88 v30,73.88 | v31,73.88 31,75 D1.C | v32,73.88 32,75
  other vias: 27.24,36.8
  pour Route3 (isolate 0.1): 0,85 55,85 55,0 0,0

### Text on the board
tPlace: PP | GND | INT | 7..26V | GND | +VM | GND | +5V | L | R | GND | REF1 | B2 | B1 | A2 | A1 | GND | GND | B2 | B1 | A2 | A1 | +5V | L | R | GND | GND | REF2 | TMC5041-Eval v1.1
bPlace: TMC-Evaluation-Platform: | TMC5041-Eval | Interfaces: | SPI | Voltage: | 7V...26V | Current: | 2x1.1A RMS | v1.1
